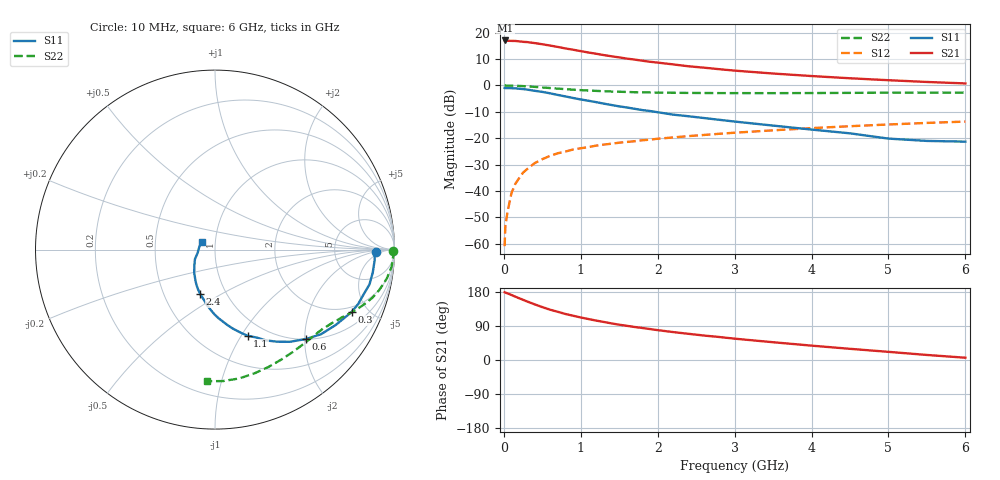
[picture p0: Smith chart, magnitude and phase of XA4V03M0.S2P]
! SIEMENS Discrete & RF Semiconductors
! BFY180
! Si NPN RF Bipolar Junction Transistor in MICRO-X
! VCE = 4 V  IC = 3 mA
! Common Emitter S-Parameters:  May  1997
# GHz  S  MA  R  50
!  f  S11  S21  S12  S22
! GHz  MAG  ANG  MAG  ANG  MAG  ANG  MAG  ANG
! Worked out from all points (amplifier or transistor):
!   36 points, 10 MHz to 6 GHz, reference 50 ohm
!   highest |S21| = 17.1 dB at 20 MHz (marker M1)
!   |S21| within 3 dB of that: start of sweep to 795.6 MHz
!   unconditionally stable (mu >= 1): 2.316 GHz to end of sweep
!   at 250 MHz: K = 0.17, MSG = 24.8 dB, |S12| = -33.0 dB
!   at 1.4 GHz: K = 0.79, MSG = 16.6 dB, |S12| = -22.1 dB
!   at 6 GHz: K = 1.07, MAG = 5.6 dB, |S12| = -13.7 dB
!   S11 on the Smith chart (normalised r, x): 10 MHz: 18, -2; 300 MHz: 1.69, -3.92; 600 MHz: 1.01, -2.03; 1.1 GHz: 0.82, -1.07; 2.4 GHz: 0.76, -0.40; 6 GHz: 0.86, +0.08
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0.01  0.8957 -0.8  7.043 178.7  0.0009 86.6  0.9926 -0.3
0.02  0.8905 -1.7  7.13 177.8  0.0022 90.9  0.9999 -0.7
0.05  0.8913 -3.9  7.018 175.7  0.0042 85.1  0.9938 -1.9
0.1  0.8882 -8.3  6.997 171.5  0.0092 86.6  0.991 -3.8
0.15  0.8823 -12.7  6.974 167.1  0.0137 83.2  0.9878 -5.7
0.3  0.8373 -24.5  6.652 154.6  0.0258 76.4  0.9618 -10.9
0.4  0.7928 -32.0  6.361 146.9  0.0337 71.7  0.9412 -14.0
0.5  0.7558 -38.6  6.042 139.6  0.0401 67.8  0.9179 -16.9
0.6  0.7106 -44.5  5.71 132.8  0.0463 64.6  0.894 -19.3
0.8  0.6199 -55.9  5.033 121.5  0.0559 60.0  0.8515 -23.3
1  0.5426 -64.6  4.477 112.2  0.0645 55.9  0.8159 -26.8
1.1  0.513 -69.3  4.214 108.1  0.068 54.6  0.8012 -28.1
1.3  0.4525 -77.1  3.765 100.4  0.0758 52.3  0.7775 -31.0
1.5  0.4015 -84.0  3.4 93.1  0.0823 50.6  0.76 -33.7
1.7  0.3613 -90.4  3.094 87.1  0.0878 49.2  0.7448 -36.2
2.2  0.28 -103.8  2.508 73.7  0.1035 45.6  0.7272 -42.8
2.4  0.261 -108.4  2.312 69.1  0.1097 44.6  0.7222 -45.3
3  0.2071 -121.5  1.912 56.3  0.1272 40.7  0.7165 -52.8
3.5  0.1736 -131.9  1.684 46.9  0.1412 37.6  0.7154 -59.1
4.5  0.1238 -154.5  1.369 29.5  0.169 30.3  0.7237 -72.4
5.5  0.0889 170.8  1.165 13.3  0.1951 22.8  0.7338 -86.5
6  0.0862 149.4  1.093 6.0  0.2067 18.5  0.735 -93.6
